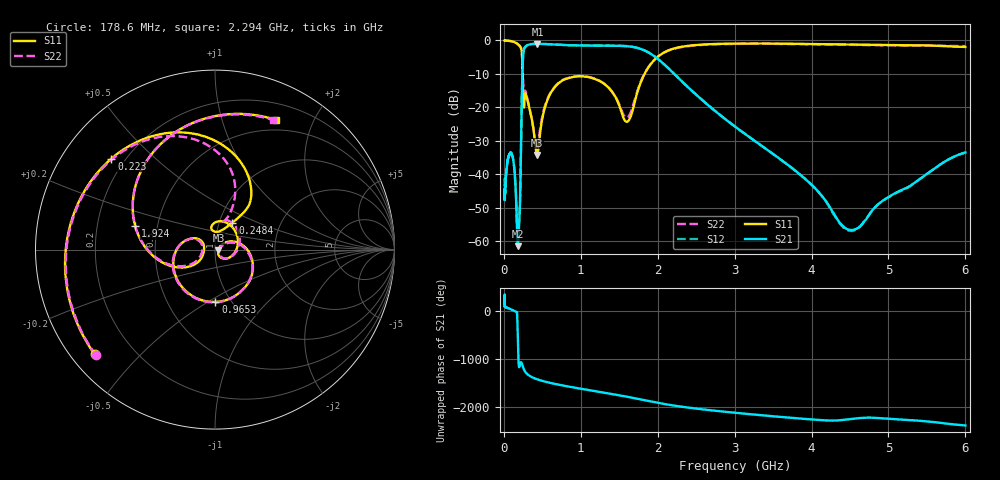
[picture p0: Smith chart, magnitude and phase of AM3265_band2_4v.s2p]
!Agilent Technologies,E8364B,MY43040894,A.07.50.67
!Agilent E8364B: A.07.50.67
!Date: Friday, May 09, 2025 07:24:10
!Correction: S11(Full 2 Port(1,2))
!S21(Full 2 Port(1,2))
!S12(Full 2 Port(1,2))
!S22(Full 2 Port(1,2))
!S2P File: Measurements: S11, S21, S12, S22:Log Frequency Sweep
# Hz S  dB  R 50
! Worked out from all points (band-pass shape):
!   3201 points, 10 MHz to 6 GHz, reference 50 ohm
!   highest |S21| = -1.01 dB at 436.5 MHz (marker M1); lowest = -61.5 dB at 183.3 MHz (marker M2)
!   |S21| within 3 dB of the highest: 252.8 MHz to 1.911 GHz (1.659 GHz wide, 153 % of centre)
!   lowest |S11| = -34.2 dB at 431.3 MHz (marker M3), VSWR 1.04, Z = 51.9 - j0.447 ohm
!   |S11| at or under -10 dB: 243.4 MHz to 1.829 GHz (1.586 GHz wide, 153 % of centre)
!   |S22| runs from -32.0 to 0.0 dB; largest |S21 - S12| = 0.014
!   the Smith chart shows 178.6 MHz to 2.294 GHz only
!   S11 on the Smith chart (normalised r, x): 178.6 MHz: 0.07, -0.37; 223 MHz: 0.15, +0.37; 248.4 MHz: 1.16, +0.36; 965.3 MHz: 0.85, -0.54; 1.924 GHz: 0.37, +0.13; 2.294 GHz: 0.38, +1.50
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1e7  -0.03 -6.2  -45.45 132.6  -41.11 -64.3  -0.05 -6.1
2.908064e7  -0.04 -17.6  -39.88 74.8  -39.83 72.8  -0.04 -17.6
8.439949e7  -0.14 -53.1  -33.59 37.5  -33.46 35.3  -0.18 -53.4
1.786094e8  -1.02 -139.0  -60.35 18.8  -58.49 173.0  -1.05 -138.5
1.833119e8  -1.11 -145.3  -61.46 74.3  -58.65 61.7  -1.13 -144.6
2.229829e8  -2.29 138.7  -31.99 10.6  -32.03 12.6  -2.25 143.3
2.44949e8  -12.00 52.6  -7.37 -66.9  -7.33 -66.9  -8.96 71.5
2.484007e8  -14.94 57.1  -5.57 -85.3  -5.53 -85.3  -11.05 68.2
3.221182e8  -19.26 -11.2  -1.26 100.0  -1.23 99.9  -19.09 -12.7
4.31289e8  -34.18 -12.7  -1.01 14.7  -0.98 14.7  -31.92 -6.6
4.364931e8  -33.98 -2.2  -1.01 11.8  -0.98 11.8  -31.65 1.1
7.123273e8  -12.77 -23.2  -1.28 -99.0  -1.25 -99.0  -12.65 -26.7
9.652544e8  -10.72 -89.5  -1.48 -173.2  -1.45 -173.2  -10.62 -92.0
1.347803e9  -13.80 175.7  -1.54 82.6  -1.51 82.6  -13.73 175.6
1.923806e9  -6.66 163.4  -4.20 -92.8  -4.17 -92.8  -6.59 162.6
2.067357e9  -3.79 121.6  -6.79 -136.2  -6.76 -136.1  -3.80 121.8
2.293826e9  -1.96 64.9  -11.79 166.2  -11.76 166.2  -2.03 65.8
3.202913e9  -0.90 -91.5  -29.06 6.0  -29.06 5.9  -0.97 -91.5
3.818953e9  -1.01 -178.2  -39.47 -80.3  -39.42 -80.6  -1.09 -179.7
4.490206e9  -1.22 92.0  -56.57 -98.5  -56.80 -91.7  -1.30 90.5
5.185309e9  -1.41 1.1  -44.53 -108.4  -44.70 -109.0  -1.52 1.3
6e9  -1.93 -96.9  -33.48 131.9  -33.51 131.9  -1.68 -96.5
